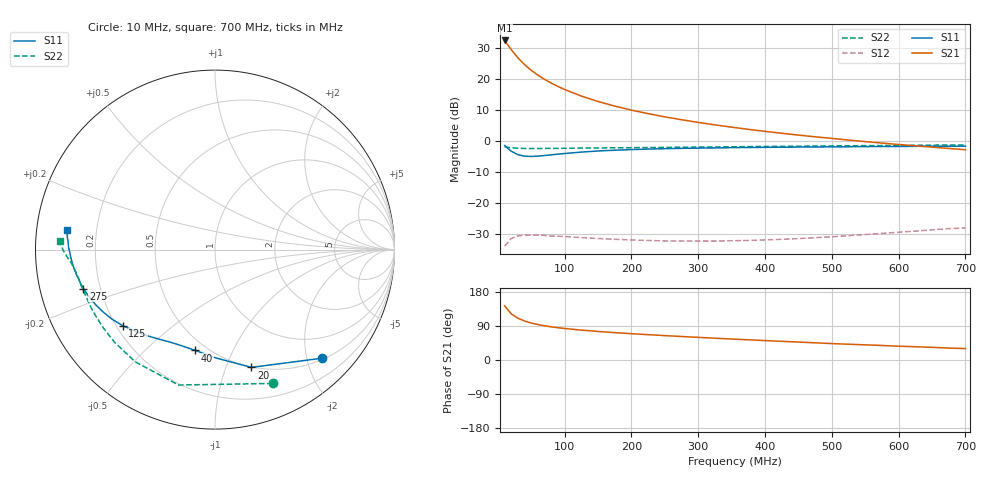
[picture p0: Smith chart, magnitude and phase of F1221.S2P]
! Date: Tue Aug 08 10:07:32 1995
# MHZ  S  MA  R  50.0000
!  POLYFET RF DEVICES
!  F1221
!  S PARAMETERS
!  VDS=12.5V, IDQ=200mA
! FREQ  S11MAG  S11ANG  S21MAG  S21ANG  S12MAG  S12ANG  S22MAG  S22ANG
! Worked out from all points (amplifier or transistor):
!   34 points, 10 MHz to 700 MHz, reference 50 ohm
!   highest |S21| = 32.4 dB at 10 MHz (marker M1)
!   |S21| within 3 dB of that: start of sweep to 20.11 MHz
!   unconditionally stable (mu >= 1): 254.1 MHz to end of sweep
!   at 60 MHz: K = 0.15, MSG = 25.8 dB, |S12| = -30.3 dB
!   at 300 MHz: K = 1.19, MAG = 16.4 dB, |S12| = -32.2 dB
!   at 700 MHz: K = 1.44, MAG = 8.7 dB, |S12| = -28.0 dB
!   S11 on the Smith chart (normalised r, x): 10 MHz: 0.53, -2.29; 20 MHz: 0.50, -1.23; 40 MHz: 0.43, -0.73; 125 MHz: 0.23, -0.34; 275 MHz: 0.14, -0.14; 700 MHz: 0.09, +0.06
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10  0.8502 -45.4  41.7 143.0  0.02035 52.1  0.812 -66.7
20  0.6869 -72.8  29.62 121.7  0.02699 34.2  0.7814 -105.1
30  0.6031 -89.7  21.83 110.1  0.02975 22.8  0.7672 -125.5
40  0.5724 -101.1  16.97 102.7  0.03047 17.1  0.7613 -137.6
50  0.5668 -109.3  13.75 97.5  0.03073 12.6  0.7601 -145.2
60  0.573 -115.9  11.51 93.5  0.0305 10.1  0.7601 -150.5
70  0.5859 -121.2  9.842 90.2  0.03029 7.8  0.7623 -154.4
80  0.6012 -125.8  8.564 87.5  0.02958 7.0  0.7628 -157.2
90  0.6171 -129.8  7.568 85.2  0.02946 5.6  0.7641 -159.6
100  0.6314 -133.2  6.759 83.2  0.02909 5.4  0.7664 -161.5
125  0.6658 -140.4  5.306 78.8  0.02794 5.1  0.7718 -164.9
150  0.6932 -146.1  4.344 75.3  0.02704 6.2  0.7751 -167.3
175  0.7137 -150.9  3.659 72.2  0.02623 7.6  0.7804 -169.1
200  0.7303 -154.7  3.152 69.4  0.02562 10.2  0.7835 -170.4
225  0.7439 -158.1  2.766 66.9  0.02517 12.4  0.788 -171.6
250  0.755 -160.9  2.455 64.4  0.02472 14.9  0.7924 -172.5
275  0.7644 -163.5  2.208 62.0  0.02471 17.8  0.7972 -173.3
325  0.7771 -167.8  1.825 57.5  0.02452 24.5  0.805 -174.8
375  0.7889 -171.3  1.546 53.3  0.02518 30.3  0.8148 -176.0
475  0.805 -177.1  1.173 45.4  0.02789 42.1  0.8321 -178.2
600  0.8199 176.8  0.882 36.4  0.03408 52.6  0.8523 179.3
700  0.8303 172.5  0.7263 30.1  0.03993 57.4  0.8672 177.0
